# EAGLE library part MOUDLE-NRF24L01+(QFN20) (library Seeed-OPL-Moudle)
113990011
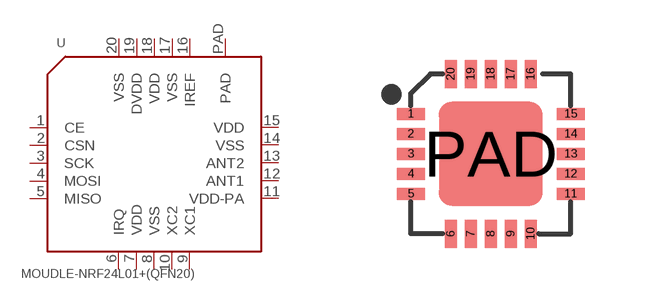
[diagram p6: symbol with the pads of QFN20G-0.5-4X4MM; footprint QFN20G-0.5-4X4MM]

Designator prefix U

## MOUDLE-NRF24L01+(QFN20) (MPN: NRF24L01+; VALUE: NRF24L01+)  [QFN20G-0.5-4X4MM]
1  CE
2  CSN
3  SCK
4  MOSI
5  MISO
6  IRQ
7  VDD
8  VSS
9  XC1
10  XC2
11  VDD-PA
12  ANT1
13  ANT2
14  VSS
15  VDD
16  IREF
17  VSS
18  VDD
19  DVDD
20  VSS
PAD  PAD

## Footprint QFN20G-0.5-4X4MM (pad centres in mm)
smd 0.7 x 0.3: 1 -2,1; 2 -2,0.5; 3 -2,0; 4 -2,-0.5; 5 -2,-1; 11 2,-1; 12 2,-0.5; 13 2,0; 14 2,0.5; 15 2,1
smd 0.3 x 0.7: 6 -1,-2; 7 -0.5,-2; 8 0,-2; 9 0.5,-2; 10 1,-2; 16 1,2; 17 0.5,2; 18 0,2; 19 -0.5,2; 20 -1,2
smd 2.6 x 2.6: PAD 0,0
